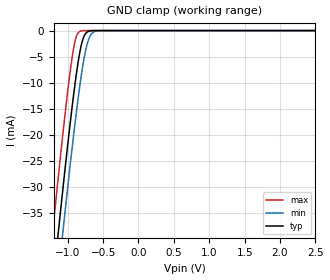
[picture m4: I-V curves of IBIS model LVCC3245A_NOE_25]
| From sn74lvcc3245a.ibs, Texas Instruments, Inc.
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[Model]   LVCC3245A_NOE_25
Model_type  Input
Vinl=0.7
Vinh=1.7
| variable   typ   min   max
C_comp   3.27pF   2.65pF   4.07pF
[Temperature Range]   40   100   -40
| Ambient temperature   25   85   -40
[Voltage range]   2.5   2.3   2.7
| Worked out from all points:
|   GND clamp passes 1 mA (typ) near -0.77 V on its own axis
[GND Clamp]
| LVCC3245A_NOE_25
|   Voltage   I(typ)   I(min)   I(max)
-5.5V     -655.9mA   -662.9mA   -647.3mA
-1.215V   -49.65mA   -57.94mA   -39mA
-1.14V    -39.76mA   -48.06mA   -29.1mA
-1.075V   -31.38mA   -39.65mA   -20.78mA
-1.06V    -29.48mA   -37.73mA   -18.91mA
-960mV    -17.27mA   -25.29mA   -7.385mA
-885mV    -9.107mA   -16.56mA   -1.488mA
-830mV    -4.286mA   -10.76mA   -171.8uA
-780mV    -1.473mA   -6.233mA   -17.17uA
-720mV    -242.8uA   -2.357mA   -1.024uA
-650mV    -22.03uA   -444.4uA   -37.97nA
2.5V      4.713pA    7.579pA    4.389pA
